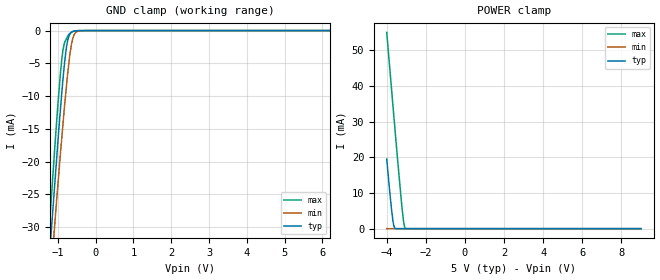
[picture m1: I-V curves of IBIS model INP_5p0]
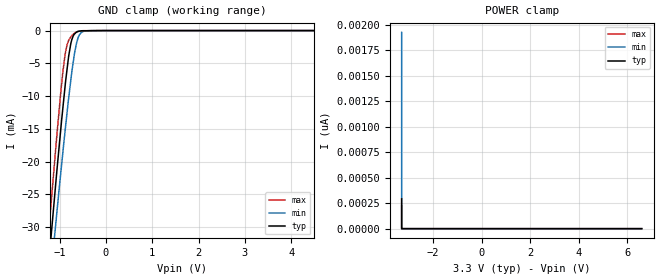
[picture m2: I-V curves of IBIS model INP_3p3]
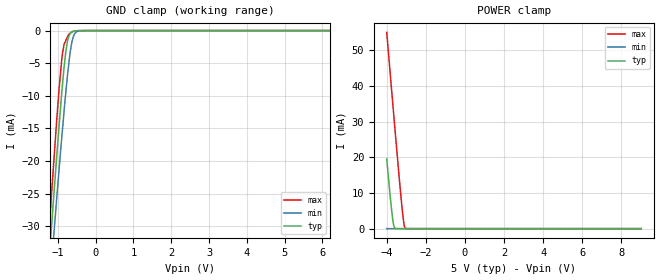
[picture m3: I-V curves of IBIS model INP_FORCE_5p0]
| TEXAS INSTRUMENTS INCORPORATED
| Standard Linear and Logic Group
| IBIS Model of TRS3243E RHB
| 3-V TO 5.5-V MULTICHANNEL RS-232 LINE DRIVER/RECEIVER WITH+/-15-kV IEC
| ESD PROTECTION
| This file contains package information for the following:
| VQFN - 32-pin (RHB) package as [Component] TRS3243E RHB
| This device can be powered at the following Vccs:
|  5 volt Vcc
|  3.3 volt Vcc
| This file provides unique models under the [Model Selector] for each Vcc.
| For operation at a specific Vcc, select the appropriate model after each
| [Model Selector] keyword.
| DOUT Models : DOUT buffer works on VPLUS and VMINUS Supply rails
|   (Chargepump Output Voltage).
|   - DOUT_5p0 Model captures the corresponding chargepump and
|   transient response of the bufer when VCC = 5V
|   - DOUT_3p3 Model captures the corresponding chargepump and
|   transient response of the bufer when VCC = 3.3V
[IBIS Ver]   3.2
[Comment char]  |_char
[File Name]   trsf3243e_rhb.ibs
[File Rev]   1.0 | x_die
[Date]   November 19, 2021
[Source]   Data created from TI-SPICE simulations at TI-SLL.
[Notes]   The following is an IBIS list for TRSF3243E RGT
[Disclaimer] Property of Texas Instruments Incorporated.  Unauthorized
   reproduction and/or distribution is strictly prohibited.
   This product is protected under copyright law.
   Created  2021, (C) Copyright  2021, Texas Instruments
   Incorporated, All Rights Reserved
   UNLESS THERE IS A SIGNED, WRITTEN AGREEMENT TO THE
   CONTRARY, TEXAS INSTRUMENTS (TI) IS PROVIDING THE IBIS
   MODELS  AND WITHOUT ANY WARRANTY, EXPRESSED OR
   IMPLIED.  TI assumes no liability for:
   1) the accuracy of the IBIS models provided to your
   company;
   2) the proper functioning of these IBIS Models in your
   design or for any resulting applications; or
   3) infringement of patents, copyrights or intellectual
   property rights resulting from your use of these IBIS
   models.
   TI provides IBIS Models as a service to our customers.
   You and your company shall not distribute, sell or give
   these models to anyone else without prior written
   permission from TI.
   TI reserves the right to make changes to our products or
   to discontinue any semiconductor product or service
   without notice, and advises our customers to obtain the
   latest version of relevant information to verify, before
   placing orders, that the information being relied on is
   current.
   Please be aware that your receipt and use of the IBIS
   information provided shall serve as acceptance of these
   terms and conditions.  If you do not accept these terms,
   you should return or destroy the IBIS models and any
   other accompanying information immediately.
| Component TRSF3243E RHB
[Component]   TRSF3243E_RHB
[Manufacturer]   Texas Instruments, Inc.
[Package]   |VQFN (RHB) 32-pin
|   typ   min   max
R_pkg   0.0m   0.0m   0.0m
L_pkg   0.0nH   0.0nH   0.0nH
C_pkg   0.0pF   0.0pF   0.0pf
[Pin]   signal_name   model_name   R_pin   L_pin   C_pin
1   RIN1   RIN   na   na   na
2   RIN2   RIN   na   na   na
3   RIN3   RIN   na   na   na
4   RIN4   RIN   na   na   na
5   RIN5   RIN   na   na   na
6   DOUT1   DOUT   na   na   na
7	DOUT2   DOUT   na   na   na
8   DOUT3   DOUT   na   na   na
9   NC   NC   na   na   na
10   DIN3   INP   na   na   na
11   DIN2   INP   na   na   na
12   DIN1   INP   na   na   na
13   ROUT5   ROUT   na   na   na
14   ROUT4   ROUT   na   na   na
15   ROUT3   ROUT   na   na   na
16   NC   NC   na   na   na
17	ROUT2	  ROUT   na   na   na
18	ROUT1	  ROUT   na   na   na
19	ROUTB2	  ROUTB   na   na   na
20	INVALIDB	  INVALIDB   na   na   na
21	FORCEOFFB	  INP_FORCEB   na   na   na
22	FORCEON	  INP_FORCE   na   na   na
23	C1N	  NC   na   na   na
24	GND	  GND   na   na   na
25	NC	  NC   na   na   na
26	VCC	  POWER   na   na   na
27	VPLUS	  NC   na   na   na
28	C1P	  NC   na   na   na
29	C2P	  NC   na   na   na
30	C2N	  NC   na   na   na
31	VMINUS	  NC   na   na   na
32	NC	  NC   na   na   na
| Model INP
[Model Selector]   INP
INP_5p0   5 volt Vcc
INP_3p3   3.3 volt Vcc
| Model INP_FORCE
[Model Selector]   INP_FORCE
INP_FORCE_5p0   5 volt Vcc
INP_FORCE_3p3   3.3 volt Vcc
| Model INP_FORCEB
[Model Selector]   INP_FORCEB
INP_FORCEB_5p0   5 volt Vcc
INP_FORCEB_3p3   3.3 volt Vcc
| Model INVALIDB
[Model Selector]   INVALIDB
INVALIDB_5p0   5 volt Vcc
INVALIDB_3p3   3.3 volt Vcc
| Model RIN
[Model Selector]   RIN
RIN_5p0   5 volt Vcc
RIN_3p3   3.3 volt Vcc
| Model ROUTB
[Model Selector]   ROUTB
ROUTB_5p0   5 volt Vcc
ROUTB_3p3   3.3 volt Vcc
| Model ROUT
[Model Selector]   ROUT
ROUT_5p0   5 volt Vcc
ROUT_3p3   3.3 volt Vcc
| Model DOUT
[Model Selector]   DOUT
DOUT_5p0   5 volt Vcc
DOUT_3p3   3.3 volt Vcc
| Models and submodels in the file (16): INP_5p0 (Input), INP_3p3 (Input), INP_FORCE_5p0 (Input), INP_FORCE_3p3 (Input), INP_FORCEB_5p0 (Input), INP_FORCEB_3p3 (Input), INVALIDB_5p0 (Output), INVALIDB_3p3 (Output), RIN_5p0 (Input), RIN_3p3 (Input), ROUT_5p0 (3-state), ROUT_3p3 (3-state), ROUTB_5p0 (3-state), ROUTB_3p3 (3-state), DOUT_5p0 (3-state), DOUT_3p3 (3-state)
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[Model]   INP_5p0
Model_type   Input
Vinl = 0.8
Vinh = 2.4
|   typ   min   max
C_comp   0.75pF   0.72pF   0.79pF
[Voltage Range]   5   4.5   5.5
[Temperature Range]   27   110   -40
[Power Clamp Reference]   5   4.5   5.5
[GND Clamp Reference]   0   0   0
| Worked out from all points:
|   GND clamp passes 1 mA (typ) near -0.71 V on its own axis
|   POWER clamp passes 1 mA (typ) near -3.64 V on its own axis
[GND Clamp]
|   Voltage   I(typ)   I(min)   I(max)
-4V       -268.4mA   -254.7mA   -282.4mA
-1.341V   -44.12mA   -48.85mA   -40.42mA
-1.22V    -34.23mA   -39.82mA   -29.65mA
-1.202V   -32.87mA   -38.52mA   -28.11mA
-1.072V   -22.72mA   -28.89mA   -17.14mA
-894.1mV  -9.453mA   -16.27mA   -4.329mA
-819.8mV  -4.816mA   -11.35mA   -1.777mA
-745.9mV  -1.667mA   -6.89mA    -952.3uA
-683.6mV  -567.4uA   -3.742mA   -437.6uA
-603.6mV  -153.3uA   -1.177mA   -132.2uA
-412.6mV  -9.898uA   -22.06uA   -3.037uA
9V        0A         0A         0A
[POWER Clamp]
|   Voltage   I(typ)   I(min)   I(max)
-4V       19.5mA     4.956uA    54.98mA
-3.888V   12.78mA    156.7nA    47.72mA
-3.745V   4.891mA    59.93nA    38.47mA
-3.685V   2.243mA    19.44nA    34.62mA
-3.639V   851.2uA    0A         31.67mA
-3.548V   40.18uA    0A         25.88mA
-3.387V   158.1nA    0A         15.76mA
-3.229V   19.52nA    0A         6.473mA
-3.14V    3.558nA    0A         2.064mA
-3.107V   0A         0A         912.6uA
-3.053V   0A         0A         113.7uA
9V        0A         0A         0A
[Model]   INP_3p3
Model_type   Input
Vinl = 0.6
Vinh = 2.4
|   typ   min   max
C_comp   0.80pF   0.77pF   0.84pF
[Voltage Range]   3.3   3   3.6
[Temperature Range]   27   110   -40
[Power Clamp Reference]   3.3   3   3.6
[GND Clamp Reference]   0   0   0
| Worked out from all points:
|   GND clamp passes 1 mA (typ) near -0.71 V on its own axis
[GND Clamp]
|   Voltage   I(typ)   I(min)   I(max)
-3.3V     -208.9mA   -199.9mA   -218.1mA
-1.26V    -37.58mA   -42.55mA   -33.08mA
-1.189V   -31.91mA   -37.3mA    -26.97mA
-1.161V   -29.65mA   -35.25mA   -24.54mA
-1.062V   -21.73mA   -28.06mA   -16.27mA
-970.9mV  -14.87mA   -21.57mA   -9.235mA
-883.5mV  -8.726mA   -15.55mA   -3.811mA
-758.1mV  -2.04mA    -7.658mA   -985.1uA
-636.2mV  -247.8uA   -2.004mA   -224.8uA
-567.4mV  -80.85uA   -610.7uA   -95.6uA
-431.9mV  -29.43uA   -35.16uA   -12.98uA
6.6V      0A         0A         0A
[POWER Clamp]
|   Voltage   I(typ)   I(min)   I(max)
-3.3V     292.1pA    1.927nA    222.9pA
-3.3V     0A         0A         0A
-3.3V     0A         0A         0A
6.6V      0A         0A         0A
[Model]   INP_FORCE_5p0
Model_type   Input
Vinl = 0.8
Vinh = 2.4
|   typ   min   max
C_comp   0.748pF	0.718pF	0.787pF
[Voltage Range]   5   4.5   5.5
[Temperature Range]   27   110   -40
[Power Clamp Reference]   5   4.5   5.5
[GND Clamp Reference]   0   0   0
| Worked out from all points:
|   GND clamp passes 1 mA (typ) near -0.72 V on its own axis
|   POWER clamp passes 1 mA (typ) near -3.64 V on its own axis
[GND Clamp]
|   Voltage   I(typ)   I(min)   I(max)
-4V       -268.4mA   -254.7mA   -282.4mA
-1.247V   -36.43mA   -41.64mA   -32.15mA
-1.198V   -32.49mA   -37.96mA   -27.82mA
-1.155V   -29.07mA   -34.84mA   -24.06mA
-1.121V   -26.4mA    -32.41mA   -21.3mA
-967.6mV  -14.68mA   -21.34mA   -8.995mA
-874.5mV  -8.129mA   -14.96mA   -3.407mA
-743.1mV  -1.592mA   -6.759mA   -949.8uA
-677.6mV  -515.9uA   -3.485mA   -417.6uA
-604.2mV  -153.1uA   -1.204mA   -133.4uA
-414.7mV  -10.78uA   -23.19uA   -3.277uA
9V        0A         0A         0A
[POWER Clamp]
|   Voltage   I(typ)   I(min)   I(max)
-4V       19.5mA     4.956uA    54.98mA
-3.762V   5.737mA    48.92nA    39.55mA
-3.7V     2.812mA    23.32nA    35.55mA
-3.651V   1.121mA    3.126nA    32.39mA
-3.614V   410.2uA    0A         30.05mA
-3.557V   55.49uA    0A         26.42mA
-3.402V   170.4nA    0A         16.71mA
-3.199V   33.29nA    0A         4.845mA
-3.128V   0A         0A         1.599mA
-3.098V   0A         0A         696.1uA
-3.043V   0A         0A         72.82uA
9V        0A         0A         0A
